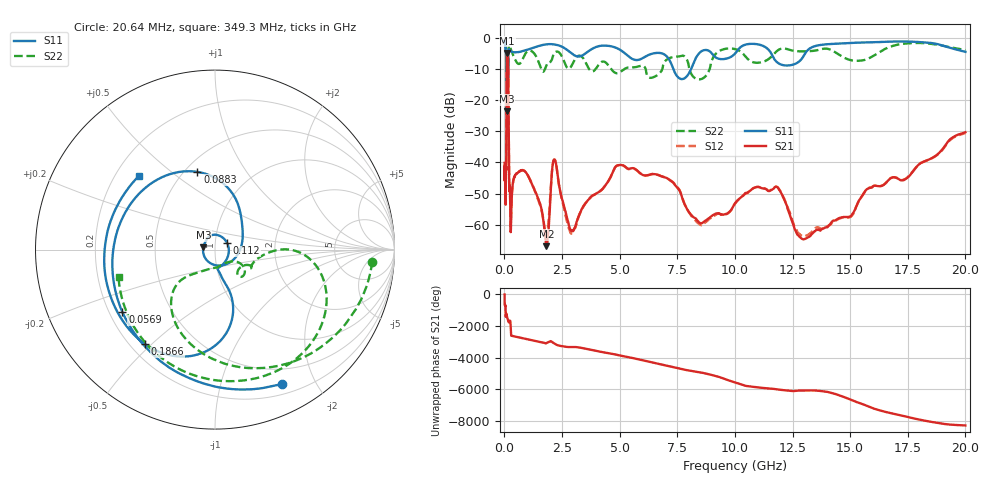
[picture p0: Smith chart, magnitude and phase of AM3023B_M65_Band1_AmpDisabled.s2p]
!Agilent Technologies,E8364B,MY43040894,A.07.50.67
!Agilent E8364B: A.07.50.67
!Date: Tuesday, October 27, 2020 10:48:20
!Correction: S11(Full 2 Port(1,2))
!S21(Full 2 Port(1,2))
!S12(Full 2 Port(1,2))
!S22(Full 2 Port(1,2))
!S2P File: Measurements: S11, S21, S12, S22:Log Frequency Sweep
# Hz S  dB  R 50
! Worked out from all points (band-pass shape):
!   3201 points, 10 MHz to 20 GHz, reference 50 ohm
!   highest |S21| = -4.90 dB at 124 MHz (marker M1); lowest = -66.9 dB at 1.82 GHz (marker M2)
!   |S21| within 3 dB of the highest: 96.6 MHz to 163.1 MHz (66.48 MHz wide, 51.2 % of centre)
!   lowest |S11| = -23.6 dB at 101.8 MHz (marker M3), VSWR 1.14, Z = 43.9 + j1.1 ohm
!   |S11| at or under -10 dB: 91.27 MHz to 161.3 MHz (70.07 MHz wide, 55.5 % of centre); 7.329 GHz to 8.103 GHz (774 MHz wide, 10 % of centre)
!   |S22| runs from -20.7 to -1.0 dB; largest |S21 - S12| = 0.014
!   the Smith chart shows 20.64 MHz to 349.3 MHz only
!   S11 on the Smith chart (normalised r, x): 20.64 MHz: 0.32, -1.57; 56.9 MHz: 0.25, -0.29; 88.3 MHz: 0.58, +0.62; 112 MHz: 1.14, +0.08; 186.6 MHz: 0.26, -0.48; 349.3 MHz: 0.30, +0.37
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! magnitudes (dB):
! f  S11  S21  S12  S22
! 10 MHz  -0.9  -40.1  -45.8  -1.0
! 20.64 MHz  -1.6  -42.1  -41.5  -1.1
! 35.55 MHz  -2.7  -41.6  -41.7  -1.5
! 56.9 MHz  -4.1  -53.2  -52.5  -2.5
! 78.78 MHz  -5.3  -41.5  -41.5  -4.8
! 88.3 MHz  -7.1  -20.0  -20.0  -9.4
! 101.8 MHz  -23.6  -6.1  -6.2  -20.0
! 112 MHz  -22.3  -5.2  -5.2  -18.1
! 124 MHz  -20.3  -4.9  -4.9  -13.4
! 126.1 MHz  -20.0  -4.9  -4.9  -13.7
! 161.8 MHz  -9.8  -7.4  -7.5  -12.4
! 186.6 MHz  -3.7  -27.2  -27.3  -2.8
! 273.5 MHz  -4.4  -62.0  -60.2  -3.6
! 349.3 MHz  -4.6  -47.9  -47.9  -5.1
! 447.2 MHz  -4.7  -44.5  -44.4  -6.7
! 1.59 GHz  -2.5  -54.4  -54.7  -10.0
! 1.82 GHz  -2.1  -66.9  -63.6  -8.8
! 2.155 GHz  -2.2  -39.1  -39.1  -5.0
! 2.907 GHz  -5.0  -61.9  -62.8  -9.1
! 5.639 GHz  -7.1  -42.0  -42.0  -9.5
! 13.17 GHz  -3.9  -64.0  -63.2  -4.3
! 20 GHz  -4.5  -30.3  -30.6  -3.9
